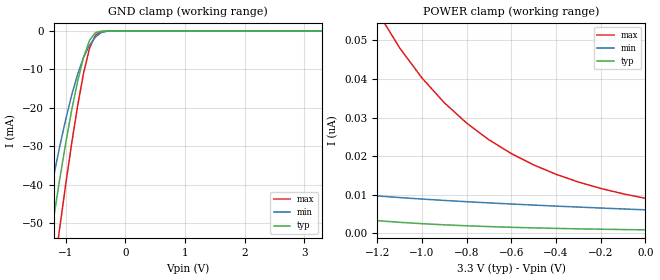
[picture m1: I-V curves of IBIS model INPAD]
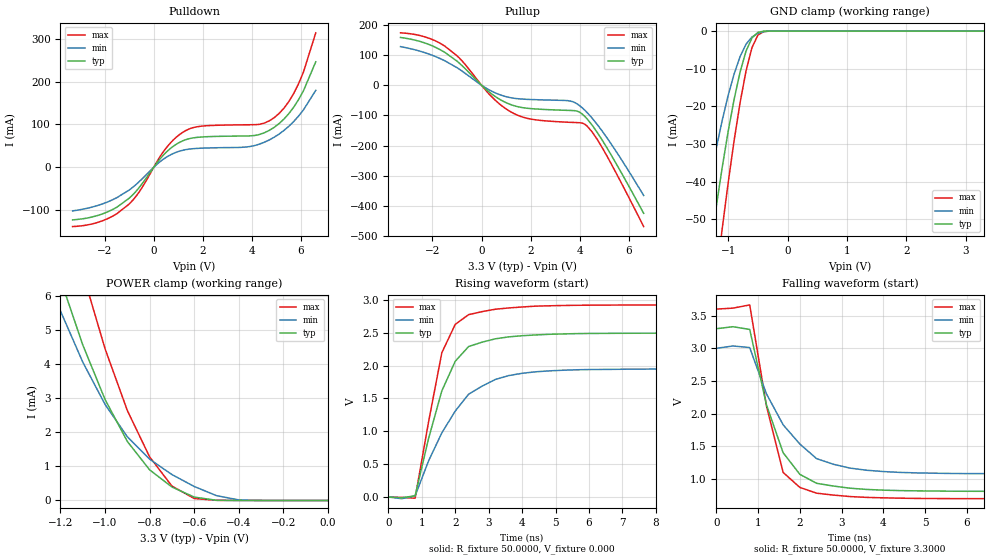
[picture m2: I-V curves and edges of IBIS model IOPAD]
| IBIS file 71v416y.ibs created by s2ibis2 version 1.1
| North Carolina State University Electronics Research Laboratory  1995
[IBIS ver]   2.1
[File name]   71v416y.ibs
[File Rev]   1.0
[Date]   10/3/03 [Filename]   71v416y.s2i
[Source]   Integrated Device Technology, Inc.
[Notes]   1. Temperatures: typ=25C, min=85C, max=0C
   2. c115_3.3v_2828_sac_speedup process.
   3. Ramp rates based on 50 ohm load.
[Copyright]   Copyright 2001, Integrated Device Technology, Inc. Integrated
   Device Technology, Inc. ("IDT") hereby grants the user of this
   IBIS model a non-exclusive, nontransferable license to use
   this IBIS model under the following terms. The user is granted
   this license only to use the IBIS model and is not granted
   rights to sell, copy (except as needed to run the IBIS model),
   rent, lease or sub-license the IBIS model in whole or in part,
   or in modified form to anyone. The User may modify the IBIS
   model to suit its specific applications, but rights to
   derivative works and such modifications shall belong to IDT.
   This IBIS model is provided on an AS IS" basis and IDT makes
   absolutely no warranty with respect to the information
   contained herein. IDT DISCLAIMS AND CUSTOMER WAIVES ALL
   WARRANTIES, EXPRESS AND IMPLIED, INCLUDING WARRANTIES OF
   MERCHANTABILITY AND FITNESS FOR A PARTICULAR PURPOSE. THE
   ENTIRE RISK AS TO QUALITY AND PERFORMANCE IS WITH THE USER
   ACCORDINGLY, IN NO EVENT SHALL IDT BE LIABLE FOR ANY DIRECT OR
   INDIRECTLY.
|   Component 71v416y
[Component]   71v416y_PH
[Manufacturer]   Integrated Device Technology
[Package]
| variable   typ   min   max
R_pkg   0.1212   0.0774   0.165
L_pkg   5.565nH   3.49nH   7.64nH
C_pkg   0.719pF   0.388pF   1.05pF
[Pin]  signal_name   model_name   R_pin   L_pin   C_pin
1   A0   INPAD   0.1343   7.64nH   0.802pF
2   A1   INPAD   0.142   6.94nH   1.05pF
3   A2   INPAD   0.148   6.27nH   0.938pF
4   A3   INPAD   0.153   5.60nH   0.823pF
5   A4   INPAD   0.158   5.00nH   0.705pF
6   NCS   INPAD   0.165   4.52nH   0.558pF
7   IO0   IOPAD   0.0782   3.76nH   0.388pF
8   IO1   IOPAD   0.0784   3.68nH   0.450pF
9   IO2   IOPAD   0.0782   3.59nH   0.428pF
10   IO3   IOPAD   0.0776   3.53nH   0.393pF
11   VDD   POWER   0.0775   3.49nH   0.385pF
12   VSS   GND   0.0774   3.51nH   0.389pF
13   IO4   IOPAD   0.0777   3.54nH   0.393pF
14   IO5   IOPAD   0.0779   3.59nH   0.428pF
15   IO6   IOPAD   0.0785   3.67nH   0.451pF
16   IO7   IOPAD   0.0783   3.76nH   0.396pF
17   NWE   INPAD   0.165   4.52nH   0.558pF
18   A5   INPAD   0.158   5.00nH   0.705pF
19   A6   INPAD   0.153   5.60nH   0.823pF
20   A7   INPAD   0.148   6.27nH   0.938pF
21   A8   INPAD   0.142   6.94nH   1.05pF
22   A9   INPAD   0.1343   7.64nH   0.802pF
23   A10   INPAD   0.1343   7.64nH   0.802pF
24   A11   INPAD   0.142   6.94nH   1.05pF
25   A12   INPAD   0.148   6.27nH   0.938pF
26   A13   INPAD   0.153   5.60nH   0.823pF
27   A14   INPAD   0.158   5.00nH   0.705pF
28   NC   NC   0.165   4.52nH   0.558pF
29   IO8   IOPAD   0.0783   3.76nH   0.396pF
30   IO9   IOPAD   0.0785   3.67nH   0.451pF
31   IO10   IOPAD   0.0779   3.59nH   0.428pF
32   IO11   IOPAD   0.0777   3.54nH   0.393pF
33   VDD   POWER   0.0774   3.51nH   0.389pF
34   VSS   GND   0.0775   3.49nH   0.385pF
35   IO12   IOPAD   0.0776   3.53nH   0.393pF
36   IO13   IOPAD   0.0782   3.59nH   0.428pF
37   IO14   IOPAD   0.0784   3.68nH   0.450pF
38   IO15   IOPAD   0.0782   3.76nH   0.388pF
39   NBLE   INPAD   0.165   4.52nH   0.558pF
40   NBHE   INPAD   0.158   5.00nH   0.705pF
41   NOE   INPAD   0.153   5.60nH   0.823pF
42   A15   INPAD   0.148   6.27nH   0.938pF
43   A16   INPAD   0.142   6.94nH   1.05pF
44   A17   INPAD   0.1343   7.64nH   0.802pF
| Models and submodels in the file (2): INPAD (Input), IOPAD (I/O)
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|   Model INPAD
[Model]   INPAD
Model_type   Input
Polarity   Non-Inverting
Vinl = 0.800V
Vinh = 2.000V
C_comp   1.94pF   1.48pF   2.40pF
[Temperature Range]   25.0000   85.0000   0.000
[Voltage Range]   3.3000V   3.0000V   3.6000V
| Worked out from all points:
|   GND clamp passes 1 mA (typ) near -0.53 V on its own axis
[GND_clamp]
| voltage   I(typ)   I(min)   I(max)
-3.3V     -298.9mA   -255.3mA   -333.3mA
-1.4V     -69.7mA    -54.31mA   -87.56mA
-1.3V     -58.86mA   -45.72mA   -75.14mA
-1.2V     -48.42mA   -37.58mA   -62.98mA
-1.1V     -38.48mA   -29.97mA   -51.19mA
-900mV    -20.6mA    -16.66mA   -29.21mA
-800mV    -13.04mA   -11.21mA   -19.42mA
-700mV    -6.798mA   -6.816mA   -10.9mA
-600mV    -2.397mA   -3.628mA   -4.387mA
-500mV    -380.7uA   -1.513mA   -1.052mA
-300mV    -1.989uA   -24.86uA   -10.73uA
3.3V      913.5pA    6.81nA     6.523nA
[POWER_clamp]
| voltage   I(typ)   I(min)   I(max)
-3.3V     85.94nA    54.73nA    2.314uA
-3V       54.74nA    39.34nA    1.422uA
-2.7V     34.4nA     28.77nA    859.8nA
-2.4V     21.37nA    21.59nA    511.5nA
-2.2V     15.5nA     18.16nA    358.7nA
-1.9V     9.562nA    14.45nA    208.4nA
-1.2V     3.289nA    9.701nA    57.56nA
-1.1V     2.867nA    9.277nA    48.09nA
-900mV    2.215nA    8.533nA    33.86nA
-700mV    1.752nA    7.894nA    24.24nA
-400mV    1.288nA    7.064nA    15.31nA
0V        913.5pA    6.096nA    9.08nA
|   Model IOPAD
[Model]   IOPAD
Model_type   I/O
Polarity   Inverting
Enable   Active-High
Vinl = 0.800V
Vinh = 2.000V
Vmeas =   1.500V
Vref = 1.50   | AC Test Load as shown
Rref = 50.00   | in the datasheet
Cref = 30.00
C_comp   2.15pF   2.00pF   2.31pF
[Temperature Range]   25.0000   85.0000   0.000
[Voltage Range]   3.3000V   3.0000V   3.6000V
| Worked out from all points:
|   slope of the pulldown table from 0 to 0.495 V, typ, clamps not added: 14.4 ohm
|   slope of the pullup table from 0 to 0.495 V, typ, clamps not added: 14.6 ohm
|   GND clamp passes 1 mA (typ) near -0.54 V on its own axis
|   POWER clamp passes 1 mA (typ) near -0.81 V on its own axis
|   rising waveform, R_fixture 50.0000, V_fixture 0.000: 20-80 % time 916ps typ, 1.31ns min, 723ps max; typ from 0 V to 2.49 V
|   falling waveform, R_fixture 50.0000, V_fixture 3.3000: 20-80 % time 744ps typ, 1.1ns min, 563ps max; typ from 3.3 V to 0.812 V
[Pulldown]
| voltage   I(typ)   I(min)   I(max)
-3.3V     -122.3mA   -101.3mA   -137.9mA
-2.1V     -108.7mA   -85.4mA    -124.7mA
-1V       -71.97mA   -52.87mA   -85.48mA
-600mV    -47.64mA   -33.83mA   -58.09mA
500mV     34.75mA    23.13mA    44.54mA
1.3V      64.4mA     41.31mA    85.55mA
2V        70.97mA    44.91mA    96.35mA
3.9V      73.32mA    48.44mA    99.34mA
4.9V      93.01mA    70.04mA    115.5mA
5.5V      125mA      95.62mA    153.1mA
5.9V      157.9mA    119.5mA    194.9mA
6.6V      246mA      179.5mA    313.5mA
[Pullup]
| voltage   I(typ)   I(min)   I(max)
-3.3V     158.4mA    127.9mA    173.8mA
-2.3V     139.9mA    107.7mA    160.2mA
-1.5V     109.2mA    81.23mA    129.9mA
-800mV    65.41mA    47.27mA    81.27mA
400mV     -28.13mA   -19.17mA   -37.17mA
1.3V      -67.22mA   -42.9mA    -93mA
2.1V      -78mA      -47.53mA   -113.4mA
3.6V      -83.52mA   -52.11mA   -122.9mA
4V        -89.78mA   -68.18mA   -124.3mA
4.3V      -111.7mA   -90.67mA   -135.6mA
5.1V      -206.9mA   -173.6mA   -233.9mA
6.6V      -424.5mA   -365.4mA   -468.5mA
[GND_clamp]
| voltage   I(typ)   I(min)   I(max)
-3.3V     -334mA     -271.1mA   -382.6mA
-1.5V     -81.65mA   -57.2mA    -107mA
-1.4V     -69.44mA   -47.93mA   -92.74mA
-1.3V     -57.72mA   -39.21mA   -78.82mA
-1.2V     -46.61mA   -31.11mA   -65.36mA
-1.1V     -36.2mA    -23.7mA    -52.47mA
-900mV    -18.14mA   -11.41mA   -29.1mA
-800mV    -10.92mA   -6.807mA   -19.08mA
-700mV    -5.358mA   -3.508mA   -10.65mA
-600mV    -1.843mA   -1.575mA   -4.427mA
-500mV    -347uA     -636.8uA   -1.085mA
3.3V      904.3pA    813.1nA    6.356nA
[POWER_clamp]
| voltage   I(typ)   I(min)   I(max)
-3.3V     98.94mA    77.82mA    120.3mA
-1.3V     8.714mA    7.283mA    12.19mA
-1.2V     6.486mA    5.555mA    9.249mA
-1.1V     4.561mA    4.057mA    6.663mA
-1V       2.962mA    2.817mA    4.449mA
-900mV    1.731mA    1.869mA    2.638mA
-800mV    898.8uA    1.211mA    1.279mA
-700mV    395.7uA    760.6uA    423.5uA
-600mV    99.87uA    411.1uA    58.89uA
-500mV    5.946uA    141.9uA    4.096uA
-400mV    186.8nA    17.22uA    290.2nA
0V        904.3pA    4.895nA    8.848nA
[Ramp]
| variable   typ   min   max
dV/dt_r   1.4958/0.8914n   1.1682/1.3220n   1.7532/0.6749n
dV/dt_f   1.4928/0.7652n   1.1508/1.1469n   1.7400/0.5660n
R_load = 50.0000
[Rising Waveform]
R_fixture = 50.0000
V_fixture = 0.000
| time   V(typ)   V(min)   V(max)
0s        0V         0V         0V
800ps     18.18mV    15.78mV    -17.73mV
1.2ns     884.5mV    546.6mV    1.137V
1.6ns     1.616V     976.4mV    2.196V
2ns       2.065V     1.307V     2.626V
2.4ns     2.289V     1.564V     2.774V
3.2ns     2.406V     1.788V     2.857V
3.6ns     2.436V     1.847V     2.876V
5.2ns     2.48V      1.928V     2.913V
20ns      2.493V     1.947V     2.922V
[Falling Waveform]
R_fixture = 50.0000
V_fixture = 3.3000
V_fixture_min = 3.0000
V_fixture_max = 3.6000
| time   V(typ)   V(min)   V(max)
0s        3.3V       3V         3.6V
400ps     3.33V      3.036V     3.615V
800ps     3.289V     3.011V     3.664V
1.2ns     2.137V     2.304V     2.121V
1.6ns     1.403V     1.83V      1.101V
2ns       1.072V     1.536V     872.5mV
2.4ns     935.7mV    1.313V     784.4mV
3.2ns     860.6mV    1.168V     732.6mV
4.8ns     819.9mV    1.095V     703.9mV
20ns      812mV      1.082V     700mV
